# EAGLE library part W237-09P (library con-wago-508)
WAGO SREW CLAMP
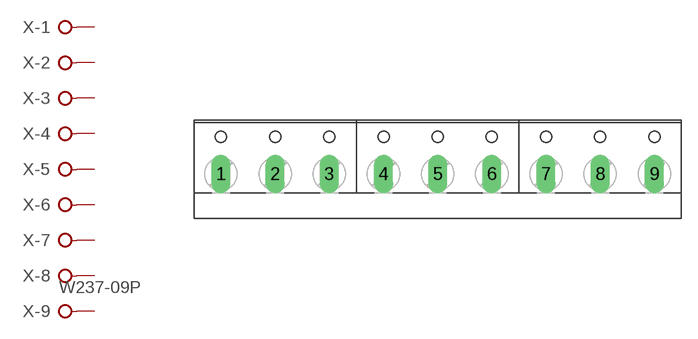
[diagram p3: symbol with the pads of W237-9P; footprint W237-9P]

Designator prefix X; gates -1=KL -2=KL -3=KL -4=KL -5=KL -6=KL -7=KL -8=KL -9=KL+V

## W237-09P (OC_FARNELL: unknown; OC_NEWARK: unknown)  [W237-9P]
1  -1:KL  pas
2  -2:KL  pas
3  -3:KL  pas
4  -4:KL  pas
5  -5:KL  pas
6  -6:KL  pas
7  -7:KL  pas
8  -8:KL  pas
9  -9:KL  pas

## Footprint W237-9P (pad centres in mm)
WAGO SREW CLAMP
drill 1.194 long: 1 -20.32,-0.635; 2 -15.24,-0.635; 3 -10.16,-0.635; 4 -5.08,-0.635; 5 0,-0.635; 6 5.08,-0.635; 7 10.16,-0.635; 8 15.24,-0.635; 9 20.32,-0.635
